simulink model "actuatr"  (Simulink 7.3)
settings: Solver=ode45  StartTime=0.0  StopTime=10.0  RelTol=1e-3

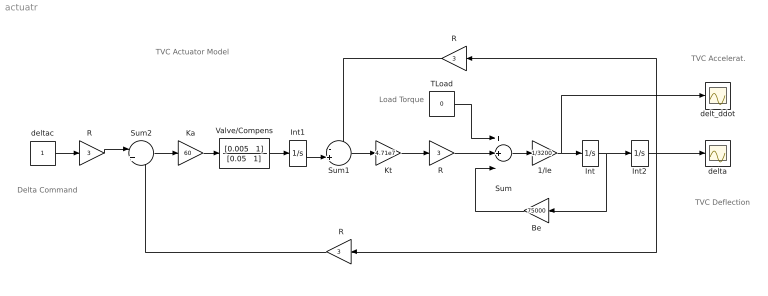
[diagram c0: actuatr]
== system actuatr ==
  note: TVC Actuator Model
  note: Delta Command
  note: TVC Deflection
  note: TVC Accelerat.
  note: Load Torque
  "  R" : Gain  Gain=3  ParameterDataType=fixdt(1, 16)  ParameterScaling=2^0  OutDataType=fixdt(1, 16)  OutScaling=2^0
  1/Ie : Gain  Gain=1/3200  ParameterDataType=fixdt(1, 16)  ParameterScaling=2^0  OutDataType=fixdt(1, 16)  OutScaling=2^0
  Be : Gain  Gain=75000  ParameterDataType=fixdt(1, 16)  ParameterScaling=2^0  OutDataType=fixdt(1, 16)  OutScaling=2^0
  Int : Integrator
  Int1 : Integrator
  Int2 : Integrator
  Ka : Gain  Gain=60  ParameterDataType=fixdt(1, 16)  ParameterScaling=2^0  OutDataType=fixdt(1, 16)  OutScaling=2^0
  Kt : Gain  Gain=4.71e7  ParameterDataType=fixdt(1, 16)  ParameterScaling=2^0  OutDataType=fixdt(1, 16)  OutScaling=2^0
  R : Gain  Gain=3  ParameterDataType=fixdt(1, 16)  ParameterScaling=2^0  OutDataType=fixdt(1, 16)  OutScaling=2^0
  "R " : Gain  Gain=3  ParameterDataType=fixdt(1, 16)  ParameterScaling=2^0  OutDataType=fixdt(1, 16)  OutScaling=2^0
  "R  " : Gain  Gain=3  ParameterDataType=fixdt(1, 16)  ParameterScaling=2^0  OutDataType=fixdt(1, 16)  OutScaling=2^0
  Sum : Sum  Inputs=++-  OutDataType=fixdt(1, 16)  OutScaling=2^0
  Sum1 : Sum  Inputs=-+|  OutDataType=fixdt(1, 16)  OutScaling=2^0
  Sum2 : Sum  Inputs=|+-  OutDataType=fixdt(1, 16)  OutScaling=2^0
  TLoad : Constant  Value=0  OutDataType=fixdt(1, 16)  OutScaling=2^0
  Valve/Compens : TransferFcn  Numerator="[0.005   1]"  Denominator="[0.05   1]"
  delt_ddot : Scope
  delta : Scope
  deltac : Constant  OutDataType=fixdt(1, 16)  OutScaling=2^0
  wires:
  Int/1 -> Int2/1, Be/1
  1/Ie/1 -> Int/1, delt_ddot/1
  Sum/1 -> 1/Ie/1
  Int2/1 -> R/1, "  R"/1, delta/1
  "R "/1 -> Sum/2
  Kt/1 -> "R "/1
  Sum1/1 -> Kt/1
  R/1 -> Sum1/1
  Be/1 -> Sum/3
  Int1/1 -> Sum1/2
  Ka/1 -> Valve/Compens/1
  "R  "/1 -> Sum2/1
  Sum2/1 -> Ka/1
  "  R"/1 -> Sum2/2
  Valve/Compens/1 -> Int1/1
  deltac/1 -> "R  "/1
  TLoad/1 -> Sum/1
